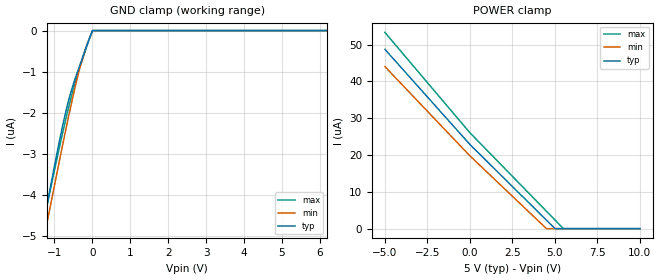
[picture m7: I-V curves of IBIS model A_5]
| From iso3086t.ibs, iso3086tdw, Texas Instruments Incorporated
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|   A_5 Model
[Model]   A_5
Model_type   Input
|Signals   A   positive pin
|Rref = 27   Note: 54 Ohm differential load;
Vinl   = 1.5V
Vinh   = 3.5V
|Rref_Diff   = 96kOhms   |Input Diff resistance
|Cref_Diff   = 7pF   |Input Diff capacitance
|Vdiff can be <= -200mV or >=-100mV and Common mode can be betweem -7V to 12V
| C_comp
|   typ   min   max
|   (Nom PVT)   (Slow PVT)   (Fast PVT)
C_comp   1.0130724pF  1.0130723pF  1.0130724pF
[Model Spec]
Vinl   1.5V   1.35V   1.65V
Vinh   3.5V   3.15V   3.85V
[Voltage Range]   5   4.5   5.5
[Temperature Range]   40   125   -40
[Power Clamp Reference]   5   4.5   5.5
[GND Clamp Reference]   0   0   0
[GND Clamp]
|   Voltage   I(typ)   I(min)   I(max)
-5V       -23.77uA   -23.05uA   -24.37uA
-1.377V   -5.139uA   -5.531uA   -5.071uA
-1.272V   -4.618uA   -5.036uA   -4.595uA
-1.235V   -4.433uA   -4.86uA    -4.428uA
-875mV    -2.716uA   -3.193uA   -2.868uA
-747.5mV  -2.161uA   -2.618uA   -2.343uA
-642.5mV  -1.753uA   -2.156uA   -1.929uA
-470mV    -1.214uA   -1.435uA   -1.313uA
-305mV    -773.3nA   -826.1nA   -818.5nA
-132.5mV  -322.2nA   -315.3nA   -341nA
2.5mV     0A         0A         0A
10V       0A         0A         0A
[POWER Clamp]
|   Voltage   I(typ)   I(min)   I(max)
-5V       48.71uA    44.02uA    53.3uA
2.5mV     22.84uA    19.75uA    26.02uA
4.503V    2.294uA    0A         4.721uA
5.005V    0A         0A         2.343uA
5.5V      0A         0A         0A
10V       0A         0A         0A
